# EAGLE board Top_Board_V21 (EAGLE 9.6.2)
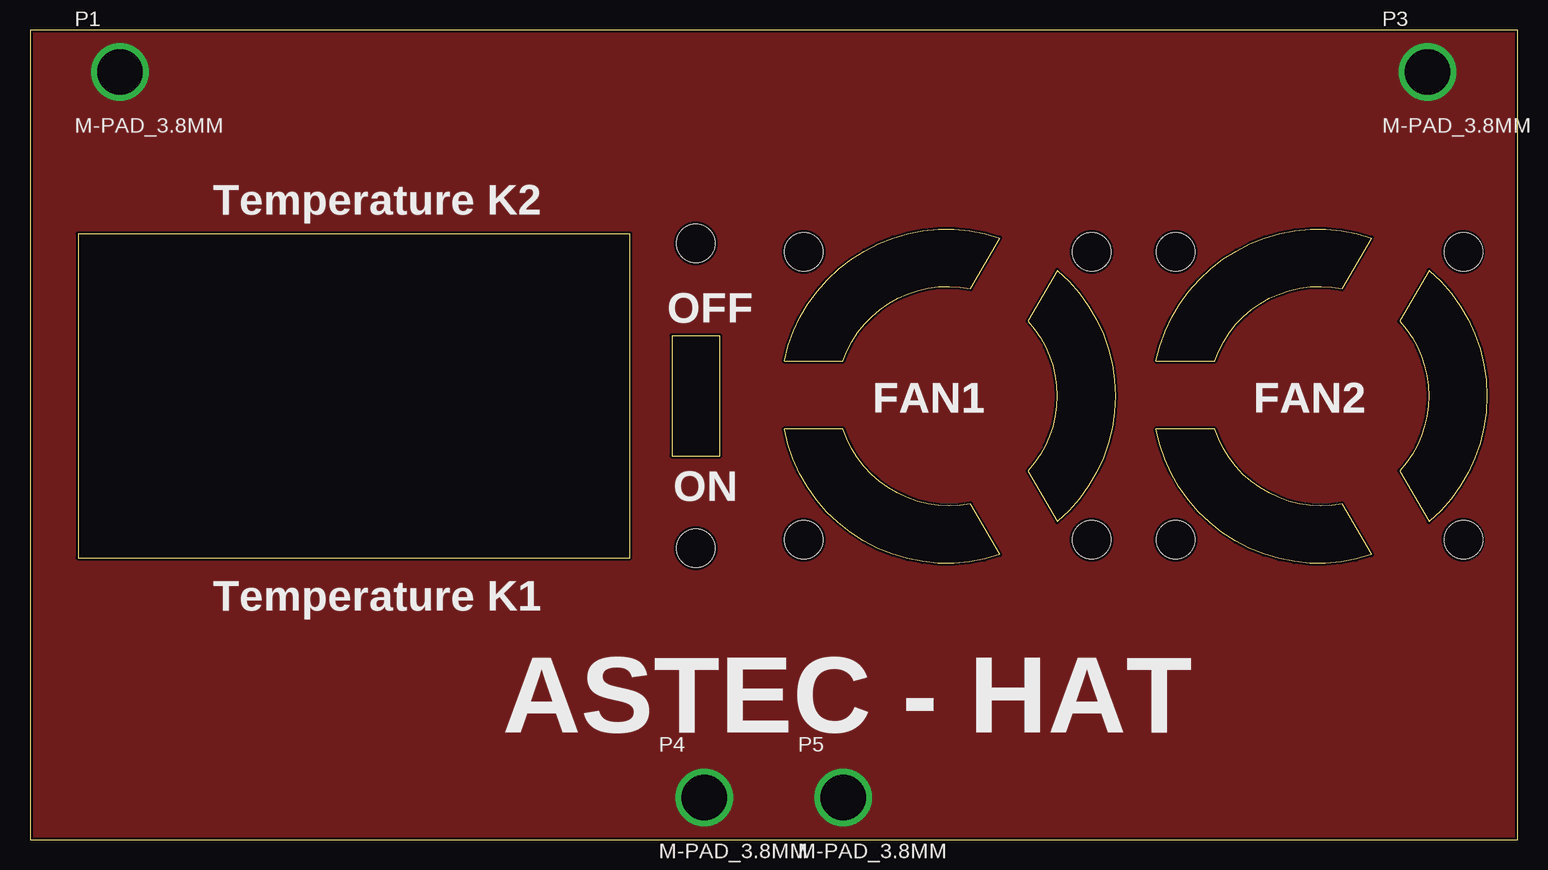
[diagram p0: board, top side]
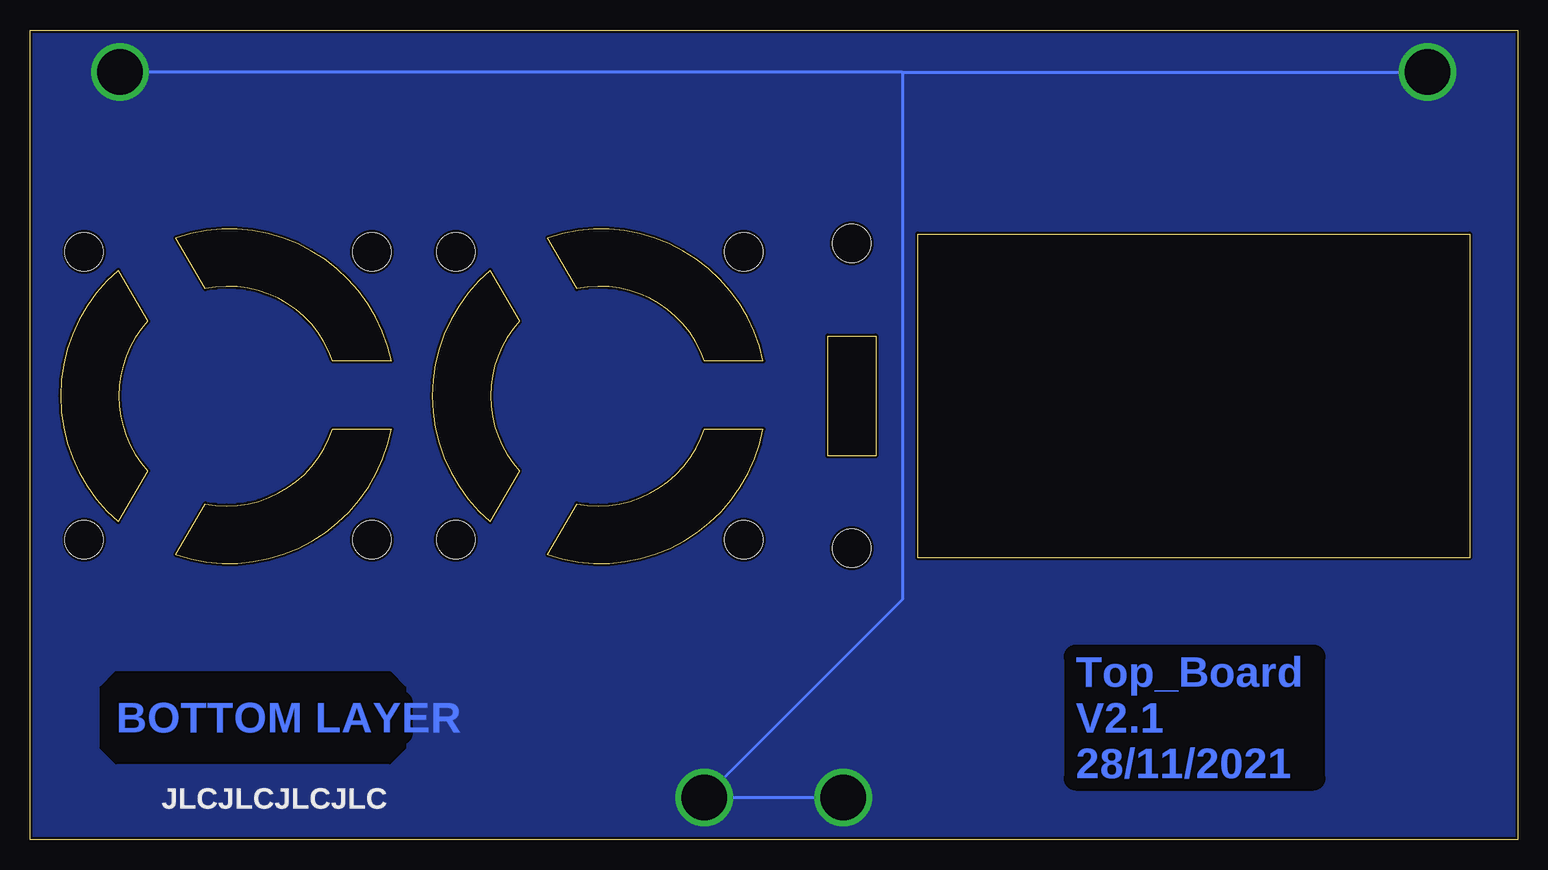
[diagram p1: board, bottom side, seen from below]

Size 124 x 67.5 mm. Coordinates in mm from the lower left corner, seen from the top.
Outline: 0,0 124,0 124,67.5 0,67.5 0,0
Outline: 4,23.5 50,23.5 50,50.5 4,50.5 4,23.5
Outline: 53.5,42 53.5,32 57.5,32 57.5,42 53.5,42
Outline: 62.88,39.9 67.78,39.9 arc-83 78.4,45.92 80.85,50.16 arc97 62.88,39.9
Outline: 80.85,23.75 78.4,28 arc-83 67.78,34.23 62.88,34.23 arc98 80.85,23.75
Outline: 85.64,47.45 83.19,43.21 arc-85 83.19,30.75 85.64,26.51 arc99 85.64,47.45
Outline: 93.87,39.9 98.77,39.9 arc-83 109.39,45.92 111.84,50.16 arc97 93.87,39.9
Outline: 111.84,23.75 109.39,28 arc-83 98.77,34.23 93.87,34.23 arc98 111.84,23.75
Outline: 116.63,47.45 114.18,43.21 arc-85 114.18,30.75 116.63,26.51 arc99 116.63,47.45
Copper layers (1*16): Top 0.035mm / dielectric 1.5mm / Bottom 0.035mm
Design rules "JLCPCB_2alyer": minimum track width 5mil, minimum drill 0.2mm, track to track 5mil, track to pad 0.2mm, pad to pad 0.2mm, via to via 0.2mm, smd to smd 5mil, copper to edge 0.2mm, drill to drill 0.5mm, minimum pad ring 0.13mm, minimum via ring 0.13mm, stop-mask expansion 0.05mm, vias tented up to drill 0mil, thermal gap 10mil
Net classes: 1 Versorgung: clearance 1 mm
Holes 3.2 mm at 55.5,49.7 55.5,24.3 64.5,25 88.5,25 95.5,25 95.5,49 88.5,49 64.5,49 119.49,25 119.49,49
bRestrict: 8 lines
Milling: 32 lines

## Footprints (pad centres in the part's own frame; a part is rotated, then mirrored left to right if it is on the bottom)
M-PAD_3.8MM = drill 3.8 pad 4.4: P$1 0,0

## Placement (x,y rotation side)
P1  M-PAD_3.8MM  [M-PAD_3.8MM]  7.5,64 0 top
P3  M-PAD_3.8MM  [M-PAD_3.8MM]  116.5,64 0 top
P4  M-PAD_3.8MM  [M-PAD_3.8MM]  56.2,3.5 0 top
P5  M-PAD_3.8MM  [M-PAD_3.8MM]  67.8,3.5 0 top

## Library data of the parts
P1 P3-P5 = Antec-Hood

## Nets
GND [Versorgung]: P1.P$1 P3.P$1 P4.P$1 P5.P$1

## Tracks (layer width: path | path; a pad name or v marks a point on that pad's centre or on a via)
GND
  Bottom 0.254: 51.29,64 P3.P$1 | P4.P$1 P5.P$1 51.29,20.01 51.29,64 | 51.29,64 P1.P$1
  pour Bottom (no thermals): -1.27,68.58 -1.27,-2.54 0,-3.81 127,-3.81 127,69.85 125.73,71.12 1.27,71.12
  pour Top (no thermals): -2.54,71.12 -2.54,-3.81 -1.27,-5.08 125.73,-5.08 127,-3.81 127,69.85 123.19,73.66 -1.27,73.66 -2.54,72.39

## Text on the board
Bottom: BOTTOM LAYER | Top_Board / V2.1 / 28/11/2021
tPlace: Temperature K2 | OFF | FAN1 | FAN1 | FAN2 | FAN2 | ON | Temperature K1 | ASTEC - HAT
bPlace: JLCJLCJLCJLC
